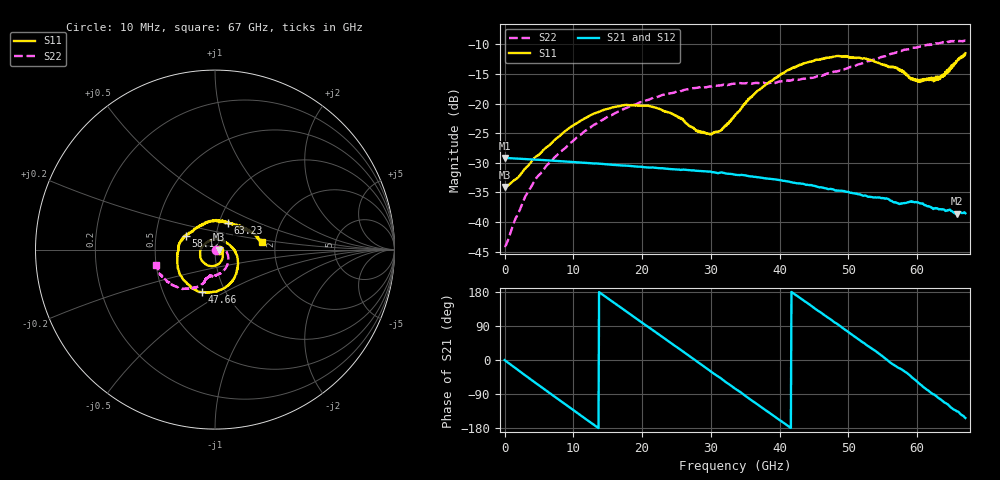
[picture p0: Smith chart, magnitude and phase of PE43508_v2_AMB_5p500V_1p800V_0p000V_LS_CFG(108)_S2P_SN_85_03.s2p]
!Keysight Technologies,N5227A,US51270237,A.10.43.00
!Date: Wednesday, August 22, 2018 17:17:57
!Correction: S11(Full 2 Port(1,3))
!S31(Full 2 Port(1,3))
!S13(Full 2 Port(1,3))
!S33(Full 2 Port(1,3))
!S2P File: Measurements: S11, S31, S13, S33:
# Hz S  dB  R 50
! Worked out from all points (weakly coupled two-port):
!   801 points, 10 MHz to 67 GHz, reference 50 ohm
!   highest |S21| = -29.16 dB at 10 MHz (marker M1); lowest = -38.6 dB at 65.74 GHz (marker M2)
!   lowest |S11| = -34.1 dB at 93.74 MHz (marker M3), VSWR 1.04, Z = 52 + j0.00589 ohm
!   |S11| at or under -10 dB: start of sweep to end of sweep
!   |S22| runs from -44.1 to -9.4 dB; largest |S21 - S12| = 0.00019
!   S11 on the Smith chart (normalised r, x): 10 MHz: 1.04, -0.00; 47.66 GHz: 0.78, -0.39; 58.12 GHz: 0.71, +0.11; 63.23 GHz: 1.10, +0.34; 67 GHz: 1.70, +0.15
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1e7  -33.97 -0.9  -29.16 -0.3  -29.16 -0.2  -44.00 -1.6
9.37375e7  -34.05 0.2  -29.17 -1.4  -29.18 -1.4  -44.05 3.8
2.940812e9  -31.04 -1.9  -29.36 -39.7  -29.36 -39.7  -35.87 34.4
4.531825e9  -28.99 -9.2  -29.46 -60.7  -29.47 -60.7  -32.74 30.7
7.3789e9  -26.03 -30.4  -29.66 -98.1  -29.66 -98.0  -28.97 19.5
1.123082e10  -22.77 -61.6  -29.95 -148.2  -29.95 -148.2  -25.08 -2.5
1.74274e10  -20.27 -111.7  -30.45 131.7  -30.45 131.7  -20.87 -34.2
2.236791e10  -20.83 -154.8  -30.89 68.1  -30.89 68.0  -18.82 -56.6
2.973681e10  -25.15 97.0  -31.48 -26.7  -31.47 -26.6  -17.11 -82.2
3.132782e10  -24.62 63.7  -31.66 -46.6  -31.66 -46.7  -16.93 -87.0
3.3505e10  -22.08 24.2  -31.99 -75.4  -31.99 -75.5  -16.65 -92.7
3.836178e10  -16.51 -31.0  -32.68 -137.2  -32.69 -137.2  -16.59 -100.7
4.162754e10  -14.14 -58.9  -33.25 -179.3  -33.25 -179.3  -16.14 -103.5
4.472582e10  -12.88 -83.7  -33.79 141.1  -33.79 141.2  -15.67 -105.7
4.765664e10  -12.15 -106.5  -34.46 103.6  -34.43 103.6  -14.74 -108.3
5.234594e10  -12.39 -144.0  -35.52 43.5  -35.50 43.4  -13.06 -113.6
5.586291e10  -13.87 -179.3  -36.17 -3.9  -36.13 -4.2  -11.73 -122.8
5.812382e10  -14.94 155.1  -36.78 -29.7  -36.80 -30.1  -10.94 -129.5
6.004979e10  -15.96 122.3  -36.65 -58.1  -36.62 -58.3  -10.53 -136.4
6.323181e10  -15.53 64.4  -37.80 -101.6  -37.84 -102.0  -9.82 -149.1
6.574394e10  -12.95 23.9  -38.58 -135.5  -38.64 -135.8  -9.47 -158.9
6.7e10  -11.51 8.7  -38.51 -153.0  -38.59 -153.0  -9.38 -165.2
